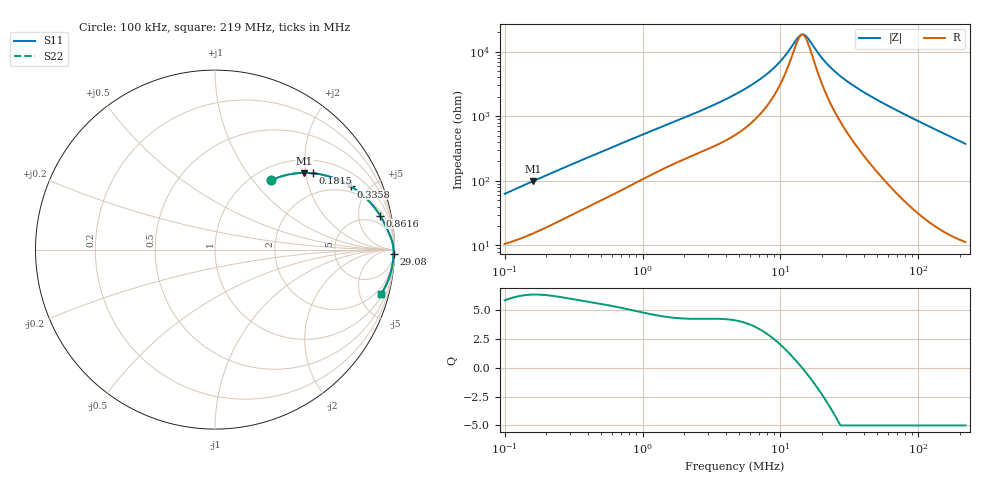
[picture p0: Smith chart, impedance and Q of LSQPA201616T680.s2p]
! LSQPA201616T680  S-PARAMETER MODEL  ( General Type )
! Model Generated by TAIYO YUDEN Corporation (http://www.ty-top.com)
! Version 2.0
! TAIYO YUDEN Control No. 100810NF25SB-FKC
! Copyright(c) 2007 TAIYO YUDEN CO.,LTD. All Rights Reserved.
! Product Description (link to TY-COMPAS)
! https://ds.yuden.co.jp/TYCOMPAS/or/detail?pn=LSQPA201616T680K&u=M
! Products Name : Inductors
! Characteristics :
!  Inductance : 68 uH , SRF(min) : 10 MHz , DC Resistance(max) : 9.1 Ohm
!  Rated Current : Saturation :130 mA , Temp Rise : 130 mA (40 degC)
!  Case Size : 2.0 x 1.6 / 0.079 x 0.063 [mm/inch] , Thickness : 1.6 / 0.063 [mm/inch]
!  (Conditions: Temperature = 25 degC , DC Bias Current/Voltage = 0A / 0V)
! External Node Assignments :
!  1  o---GGG---o  2
! GND o---------o GND
! Frequency Range : 0.1MHz  -  218.972167MHz  [ 402 STEP ]
# MHz S RI R 50
! Freq[MHz].  S11 Real  S11 Imag  S21 Real  S21 Imag  S12 Real  S12 Imag  S22 Real  S22 Imag
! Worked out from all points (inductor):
!   401 points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, 100 kHz to 219 MHz, reference 50 ohm
!   read as one part in series: L = 97.8 uH near 103.9 kHz
!   highest Q = 6.37 at 161.7 kHz (marker M1), where L = 96.8 uH
!   self-resonance near 14.27 MHz
!   S11 on the Smith chart (normalised r, x): 100 kHz: 1.21, +1.24; 181.5 kHz: 1.34, +2.19; 335.8 kHz: 1.65, +3.86; 861.6 kHz: 2.79, +8.95; 29.08 MHz: 14, -74; 219 MHz: 1.23, -7.50
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0.1  0.3117 0.3857  0.6883 -0.3857  0.6883 -0.3857  0.3117 0.3857
0.161724  0.4981 0.4276  0.5019 -0.4276  0.5019 -0.4276  0.4981 0.4276
0.181501  0.5451 0.4255  0.4549 -0.4255  0.4549 -0.4255  0.5451 0.4255
0.335824  0.7581 0.3519  0.2419 -0.3519  0.2419 -0.3519  0.7581 0.3519
0.362673  0.7785 0.3384  0.2215 -0.3384  0.2215 -0.3384  0.7785 0.3384
0.861606  0.9197 0.1895  0.0803 -0.1895  0.0803 -0.1895  0.9197 0.1895
1.315317  0.949 0.1358  0.051 -0.1358  0.051 -0.1358  0.949 0.1358
2.838371  0.9775 0.0718  0.0225 -0.0718  0.0225 -0.0718  0.9775 0.0718
4.770297  0.9876 0.0427  0.0124 -0.0427  0.0124 -0.0427  0.9876 0.0427
6.614728  0.9912 0.0281  0.00879 -0.0281  0.00879 -0.0281  0.9912 0.0281
8.658159  0.993 0.0176  0.00701 -0.0176  0.00701 -0.0176  0.993 0.0176
10.294  0.9938 0.0114  0.00625 -0.0114  0.00625 -0.0114  0.9938 0.0114
13.21743  0.9945 0.00282  0.00554 -0.00282  0.00554 -0.00282  0.9945 0.00282
14.00232  0.9946 0.000871  0.00543 -0.000871  0.00543 -0.000871  0.9946 0.000871
15.12181  0.9947 -0.00173  0.00531 0.00173  0.00531 0.00173  0.9947 -0.00173
16.97108  0.9948 -0.00567  0.00518 0.00567  0.00518 0.00567  0.9948 -0.00567
21.79075  0.9949 -0.0146  0.00508 0.0146  0.00508 0.0146  0.9949 -0.0146
29.07615  0.9947 -0.0261  0.0053 0.0261  0.0053 0.0261  0.9947 -0.0261
40.31841  0.9939 -0.0419  0.00614 0.0419  0.00614 0.0419  0.9939 -0.0419
61.54953  0.991 -0.0695  0.00904 0.0695  0.00904 0.0695  0.991 -0.0695
118.3471  0.9758 -0.138  0.0242 0.138  0.0242 0.138  0.9758 -0.138
218.9722  0.9272 -0.2451  0.0728 0.2451  0.0728 0.2451  0.9272 -0.2451
